|   IBIS model for TI xxx DSP
[IBIS Ver]   5.1
[Disclaimer]   Please be aware that in the absence of a written agreement
|   Texas Instruments(TI) assumes no liability for:
|   (1) The accuracy of the IBIS models provided to your company,
|   however, the IBIS model is compliant to industry standard
|   IQ Level 2a.  Refer to IBIS Quality Section below for
|   for full details.
|   (2) The proper functioning of these Models in your design
|   or for any resulting applications
|   (3) Infringement of patents, copyrights or intellectual
|   property rights resulting from your use of these
|   models.
|   TI provides IBIS Models as a service to our customers and
|   therefore reserves the right to limit distribution of the
|   Models.  The information is subject to change without notice.
[File Name]  sprm825f.ibs
[File Rev]   1.1
|   -Initial version
|   - Removed unsupported SDIO/LVCMOS models
|   - Removed unsupported LVDS models
|   - Removed unsupported IIC and eMMC models
|   - Added LVCMOS models with stronger drive strength supported
|   - Modify default drive strength for EMMC to 50 ohms
|   - Addition of selected drive strengths for EMMC
|   - Addition of power-aware models for eMMC
|   - Updated to align with final AM62P Pkg
|   - Addition of open-drain models for eMMC
|   - Updated to include push-pull models for eMMC
|   - Removed older eMMC models and updated to include models for latest silicon revision
[Date]   16 June 2025
[Source]   Texas Instruments Incorporated
[Copyright]   Property of Texas Instruments Incorporated.
|   Unauthorized reproduction and/or distribution is strictly.
|   prohibited.
|   This product is protected under copyright law and trade
|   secret law as an unpublished work.
|   Created 2012,(C) Copyright 1999-2012,
|   Texas Instruments Incorporated., All Rights Reserved.
|   These commodities are under the U.S. Government
|   distribution license control. As such,they are not to be
|   re-exported without the prior approval of the U.S.
|   Department of Commerce.
[Notes]
   This file does not include AMI models for SerDes based links.
   For SerDes simulations use Texas Instruments IBIS AMI models
   Some IV curves contain Non monotonic data points.
|   Revision History
|   GERNERAL COMMENT: All IBIS Quality Notes below reflect latest release
|   and version of IBIS File
|   File passes ibischk5.1 and ibischk6 with 0 errors and 287 warnings
|   Component AM62P
[Component] AM62P
[Manufacturer] Texas Instruments
[Package]
|   typ   min   max
R_pkg   0.41053   0.082407   0.73268
L_pkg   2.874e-9   9.307e-10   4.887e-9
C_pkg   1.029e-12   4.145e-13   1.599e-12
[Package Model]   am62p_pkg
[Pin]	Signal_name	model_name
B5	ATEST0	NC
Y19	ATEST1	NC
Y13	CSI0_ATB_0_H	NC
Y14	CSI0_ATB_1_H	NC
AE12	CSI0_RXCLKN	NC
AE11	CSI0_RXCLKP	NC
AB11	CSI0_RXN0	NC
AC10	CSI0_RXN1	NC
AA10	CSI0_RXN2	NC
AD9	CSI0_RXN3	NC
AB10	CSI0_RXP0	NC
AC9	CSI0_RXP1	NC
AA9	CSI0_RXP2	NC
AD8	CSI0_RXP3	NC
AA15	CSI0_RXRCALIB	NC
K5	DDR0_A0	DDR_SE
L2	DDR0_A1	DDR_SE
R2	DDR0_A10	DDR_SE
N5	DDR0_A11	DDR_SE
P3	DDR0_A12	DDR_SE
P2	DDR0_A13	DDR_SE
L3	DDR0_A2	DDR_SE
M2	DDR0_A3	DDR_SE
N2	DDR0_A4	DDR_SE
K2	DDR0_A5	DDR_SE
N3	DDR0_A6	DDR_SE
L1	DDR0_A7	DDR_SE
M1	DDR0_A8	DDR_SE
T2	DDR0_A9	DDR_SE
T6	DDR0_ACT_N	DDR_SE
K3	DDR0_ALERT_N	DDR_SE
H5	DDR0_ATB0	DDR_SE
K6	DDR0_ATB1	DDR_SE
N6	DDR0_BA0	DDR_SE
K4	DDR0_BA1	DDR_SE
Y6	DDR0_BG0	DDR_SE
U6	DDR0_BG1	DDR_SE
Y5	DDR0_CAL0	DDR_SE
T5	DDR0_CAS_N	DDR_SE
R1	DDR0_CK0	DDR_DIFF_P
P1	DDR0_CK0_N	DDR_DIFF_N
N4	DDR0_CKE0	DDR_SE
P5	DDR0_CKE1	DDR_SE
L6	DDR0_CS0_N	DDR_SE
T3	DDR0_CS1_N	DDR_SE
C3	DDR0_DM0	DDR_SE
H3	DDR0_DM1	DDR_SE
V4	DDR0_DM2	DDR_SE
AD1	DDR0_DM3	DDR_SE
B2	DDR0_DQ0	DDR_SE
A3	DDR0_DQ1	DDR_SE
G5	DDR0_DQ10	DDR_SE
F2	DDR0_DQ11	DDR_SE
G3	DDR0_DQ12	DDR_SE
H4	DDR0_DQ13	DDR_SE
J2	DDR0_DQ14	DDR_SE
G2	DDR0_DQ15	DDR_SE
U2	DDR0_DQ16	DDR_SE
U3	DDR0_DQ17	DDR_SE
U5	DDR0_DQ18	DDR_SE
V5	DDR0_DQ19	DDR_SE
A4	DDR0_DQ2	DDR_SE
V2	DDR0_DQ20	DDR_SE
Y2	DDR0_DQ21	DDR_SE
Y3	DDR0_DQ22	DDR_SE
AA4	DDR0_DQ23	DDR_SE
AC2	DDR0_DQ24	DDR_SE
AA2	DDR0_DQ25	DDR_SE
AC4	DDR0_DQ26	DDR_SE
AD2	DDR0_DQ27	DDR_SE
AD3	DDR0_DQ28	DDR_SE
AC3	DDR0_DQ29	DDR_SE
A5	DDR0_DQ3	DDR_SE
AE4	DDR0_DQ30	DDR_SE
AE3	DDR0_DQ31	DDR_SE
A2	DDR0_DQ4	DDR_SE
B4	DDR0_DQ5	DDR_SE
D2	DDR0_DQ6	DDR_SE
C4	DDR0_DQ7	DDR_SE
E2	DDR0_DQ8	DDR_SE
F1	DDR0_DQ9	DDR_SE
D1	DDR0_DQS0	DDR_DIFF_P
C1	DDR0_DQS0_N	DDR_DIFF_N
J1	DDR0_DQS1	DDR_DIFF_P
H1	DDR0_DQS1_N	DDR_DIFF_N
W1	DDR0_DQS2	DDR_DIFF_P
V1	DDR0_DQS2_N	DDR_DIFF_N
AA1	DDR0_DQS3	DDR_DIFF_P
AB1	DDR0_DQS3_N	DDR_DIFF_N
L5	DDR0_ODT0	DDR_SE
V6	DDR0_ODT1	DDR_SE
T1	DDR0_PAR	DDR_SE
P6	DDR0_RAS_N	DDR_SE
AA5	DDR0_RESET0_N	DDR_SE
T4	DDR0_WE_N	DDR_SE
AA17	DSI0_ATB_0_H	NC
Y17	DSI0_ATB_1_H	NC
AA12	DSI0_TXCLKN	NC
AA13	DSI0_TXCLKP	NC
AD11	DSI0_TXN0	NC
AB13	DSI0_TXN1	NC
AC12	DSI0_TXN2	NC
AE14	DSI0_TXN3	NC
AD12	DSI0_TXP0	NC
AB14	DSI0_TXP1	NC
AC13	DSI0_TXP2	NC
AE15	DSI0_TXP3	NC
Y16	DSI0_TXRCALIB	NC
B12	EMU0	LVCMOS_V
D13	EMU1	LVCMOS_V
C25	EXT_REFCLK1	LVCMOS_V
C23	EXTINTN	IIC_V
U22	GPMC0_AD0	LVCMOS_H
U21	GPMC0_AD1	LVCMOS_H
AA25	GPMC0_AD10	LVCMOS_H
W24	GPMC0_AD11	LVCMOS_H
Y24	GPMC0_AD12	LVCMOS_H
AD25	GPMC0_AD13	LVCMOS_H
AB24	GPMC0_AD14	LVCMOS_H
AC24	GPMC0_AD15	LVCMOS_H
U20	GPMC0_AD2	LVCMOS_H
V25	GPMC0_AD3	LVCMOS_H
T20	GPMC0_AD4	LVCMOS_H
T21	GPMC0_AD5	LVCMOS_H
V24	GPMC0_AD6	LVCMOS_H
W25	GPMC0_AD7	LVCMOS_H
AC25	GPMC0_AD8	LVCMOS_H
AB25	GPMC0_AD9	LVCMOS_H
R25	GPMC0_ADVN_ALE	LVCMOS_H
U24	GPMC0_BE0N_CLE	LVCMOS_H
T24	GPMC0_BE1N	LVCMOS_H
Y25	GPMC0_CLK	LVCMOS_H
T23	GPMC0_CSN0	LVCMOS_H
U23	GPMC0_CSN1	LVCMOS_H
T22	GPMC0_CSN2	LVCMOS_H
U25	GPMC0_CSN3	LVCMOS_H
P25	GPMC0_DIR	LVCMOS_H
R24	GPMC0_OEN_REN	LVCMOS_H
AA24	GPMC0_WAIT0	LVCMOS_H
AD24	GPMC0_WAIT1	LVCMOS_H
T25	GPMC0_WEN	LVCMOS_H
P24	GPMC0_WPN	LVCMOS_H
B25	I2C0_SCL	LVCMOS_V
A24	I2C0_SDA	LVCMOS_V
C24	I2C1_SCL	LVCMOS_V
B24	I2C1_SDA	LVCMOS_V
C5	IFORCE	NC
F20	MCAN0_RX	LVCMOS_V
B23	MCAN0_TX	LVCMOS_V
G20	MCASP0_ACLKR	LVCMOS_V
F24	MCASP0_ACLKX	LVCMOS_V
G23	MCASP0_AFSR	LVCMOS_V
F25	MCASP0_AFSX	LVCMOS_V
F23	MCASP0_AXR0	LVCMOS_V
E24	MCASP0_AXR1	LVCMOS_V
E25	MCASP0_AXR2	LVCMOS_V
D25	MCASP0_AXR3	LVCMOS_V
G6	MCU_ERRORN	LVCMOS_H
E11	MCU_I2C0_SCL	IIC_V
D11	MCU_I2C0_SDA	IIC_V
D6	MCU_MCAN0_RX	LVCMOS_V
E8	MCU_MCAN0_TX	LVCMOS_V
E7	MCU_MCAN1_RX	LVCMOS_V
F8	MCU_MCAN1_TX	LVCMOS_V
A10	MCU_OSC0_XI	NC
A11	MCU_OSC0_XO	NC
H6	MCU_PORZ	RESET_H
F14	MCU_RESETSTATZ	LVCMOS_V
F11	MCU_RESETZ	LVCMOS_V
C10	MCU_SPI0_CLK	LVCMOS_V
B10	MCU_SPI0_CS0	LVCMOS_V
E10	MCU_SPI0_CS1	LVCMOS_V
B11	MCU_SPI0_D0	LVCMOS_V
D10	MCU_SPI0_D1	LVCMOS_V
B8	MCU_UART0_CTSN	LVCMOS_V
B7	MCU_UART0_RTSN	LVCMOS_V
B6	MCU_UART0_RXD	LVCMOS_V
C8	MCU_UART0_TXD	LVCMOS_V
F17	MDIO0_MDC	LVCMOS_V
F16	MDIO0_MDIO	LVCMOS_V
AC5	MMC0_CALPAD	EMMC
AA6	MMC0_CLK	EMMC
AB8	MMC0_CMD	EMMC
AC7	MMC0_DAT0	EMMC
AB7	MMC0_DAT1	EMMC
AD6	MMC0_DAT2	EMMC
AE5	MMC0_DAT3	EMMC
AE6	MMC0_DAT4	EMMC
AC6	MMC0_DAT5	EMMC
AA7	MMC0_DAT6	EMMC
AB6	MMC0_DAT7	EMMC
AD5	MMC0_DS	EMMC
J24	MMC1_CLK	SDIO_V
H20	MMC1_CMD	SDIO_V
H21	MMC1_DAT0	SDIO_V
H23	MMC1_DAT1	SDIO_V
H22	MMC1_DAT2	SDIO_V
H25	MMC1_DAT3	SDIO_V
D23	MMC1_SDCD	LVCMOS_V
D24	MMC1_SDWP	LVCMOS_V
K21	MMC2_CLK	SDIO_H
K24	MMC2_CMD	SDIO_H
K23	MMC2_DAT0	SDIO_H
K22	MMC2_DAT1	SDIO_H
L20	MMC2_DAT2	SDIO_H
L21	MMC2_DAT3	SDIO_H
J25	MMC2_SDCD	LVCMOS_H
K25	MMC2_SDWP	LVCMOS_H
AE20	OLDI0_A0N	LVDS
AD20	OLDI0_A0P	LVDS
AC19	OLDI0_A1N	LVDS
AD19	OLDI0_A1P	LVDS
AA19	OLDI0_A2N	LVDS
AB19	OLDI0_A2P	LVDS
AD18	OLDI0_A3N	LVDS
AE19	OLDI0_A3P	LVDS
AD17	OLDI0_A4N	LVDS
AD16	OLDI0_A4P	LVDS
AB17	OLDI0_A5N	LVDS
AC17	OLDI0_A5P	LVDS
AC16	OLDI0_A6N	LVDS
AC15	OLDI0_A6P	LVDS
AB16	OLDI0_A7N	LVDS
AA16	OLDI0_A7P	LVDS
AE18	OLDI0_CLK0N	LVDS
AE17	OLDI0_CLK0P	LVDS
AD15	OLDI0_CLK1N	LVDS
AD14	OLDI0_CLK1P	LVDS
P23	OSPI0_CLK	LVCMOS_H
M25	OSPI0_CSN0	LVCMOS_H
L24	OSPI0_CSN1	LVCMOS_H
L22	OSPI0_CSN2	LVCMOS_H
L23	OSPI0_CSN3	LVCMOS_H
L25	OSPI0_D0	LVCMOS_H
N24	OSPI0_D1	LVCMOS_H
N25	OSPI0_D2	LVCMOS_H
M24	OSPI0_D3	LVCMOS_H
N21	OSPI0_D4	LVCMOS_H
N22	OSPI0_D5	LVCMOS_H
P21	OSPI0_D6	LVCMOS_H
N20	OSPI0_D7	LVCMOS_H
P22	OSPI0_DQS	LVCMOS_H
N23	OSPI0_LBCLKO	LVCMOS_H
B9	PMIC_LPM_EN0	LVCMOS_V
H24	PORZ_OUT	LVCMOS_V
G24	RESET_REQZ	LVCMOS_V
G25	RESETSTATZ	LVCMOS_V
B15	RGMII1_RD0	LVCMOS_V
B16	RGMII1_RD1	LVCMOS_V
A14	RGMII1_RD2	LVCMOS_V
B14	RGMII1_RD3	LVCMOS_V
A15	RGMII1_RX_CTL	LVCMOS_V
A16	RGMII1_RXC	LVCMOS_V
A18	RGMII1_TD0	LVCMOS_V
C17	RGMII1_TD1	LVCMOS_V
A17	RGMII1_TD2	LVCMOS_V
C16	RGMII1_TD3	LVCMOS_V
B18	RGMII1_TX_CTL	LVCMOS_V
B17	RGMII1_TXC	LVCMOS_V
E19	RGMII2_RD0	LVCMOS_V
E16	RGMII2_RD1	LVCMOS_V
E17	RGMII2_RD2	LVCMOS_V
C19	RGMII2_RD3	LVCMOS_V
F19	RGMII2_RX_CTL	LVCMOS_V
D19	RGMII2_RXC	LVCMOS_V
B19	RGMII2_TD0	LVCMOS_V
A21	RGMII2_TD1	LVCMOS_V
D17	RGMII2_TD2	LVCMOS_V
A19	RGMII2_TD3	LVCMOS_V
A20	RGMII2_TX_CTL	LVCMOS_V
D16	RGMII2_TXC	LVCMOS_V
B21	SPI0_CLK	LVCMOS_V
D20	SPI0_CS0	LVCMOS_V
E20	SPI0_CS1	LVCMOS_V
B20	SPI0_D0	LVCMOS_V
C21	SPI0_D1	LVCMOS_V
C13	TCK	LVCMOS_V
E13	TDI	LVCMOS_V
C14	TDO	LVCMOS_V
F10	TEMP_DIODE_P	NC
E14	TMS	LVCMOS_V
B13	TRSTN	LVCMOS_V
A23	UART0_CTSN	LVCMOS_V
C22	UART0_RTSN	LVCMOS_V
A22	UART0_RXD	LVCMOS_V
B22	UART0_TXD	LVCMOS_V
AE8	USB0_DM	NC
AE7	USB0_DP	NC
G22	USB0_DRVVBUS	LVCMOS_V
Y8	USB0_RCALIB	NC
Y7	USB0_VBUS	NC
AE10	USB1_DM	NC
AE9	USB1_DP	NC
G21	USB1_DRVVBUS	LVCMOS_V
1K4	USB1_RCALIB	NC
Y10	USB1_VBUS	NC
1A10	VMON_1P8_SOC	NC
1A4	VMON_3P3_SOC	NC
1A6	VMON_ER_VSYS	NC
AE24	VOUT0_DATA0	LVCMOS_H
W23	VOUT0_DATA1	LVCMOS_H
W22	VOUT0_DATA10	LVCMOS_H
AE21	VOUT0_DATA11	LVCMOS_H
AD21	VOUT0_DATA12	LVCMOS_H
AC21	VOUT0_DATA13	LVCMOS_H
AA20	VOUT0_DATA14	LVCMOS_H
Y20	VOUT0_DATA15	LVCMOS_H
AA23	VOUT0_DATA2	LVCMOS_H
Y23	VOUT0_DATA3	LVCMOS_H
AB23	VOUT0_DATA4	LVCMOS_H
AD23	VOUT0_DATA5	LVCMOS_H
AC23	VOUT0_DATA6	LVCMOS_H
AE23	VOUT0_DATA7	LVCMOS_H
AE22	VOUT0_DATA8	LVCMOS_H
AC22	VOUT0_DATA9	LVCMOS_H
W21	VOUT0_DE	LVCMOS_H
AC20	VOUT0_HSYNC	LVCMOS_H
Y21	VOUT0_PCLK	LVCMOS_H
W20	VOUT0_VSYNC	LVCMOS_H
F6	VSENSE	NC
F13	WKUP_CLKOUT0	LVCMOS_V
A13	WKUP_I2C0_SCL	IIC_V
C11	WKUP_I2C0_SDA	IIC_V
A7	WKUP_LFOSC0_XI	NC
A8	WKUP_LFOSC0_XO	NC
C7	WKUP_UART0_CTSN	LVCMOS_V
C6	WKUP_UART0_RTSN	LVCMOS_V
D8	WKUP_UART0_RXD	LVCMOS_V
D7	WKUP_UART0_TXD	LVCMOS_V
A1	VSS	GND
A6	VSS	GND
A9	VSS	GND
A12	VSS	GND
A25	VSS	GND
1G1	VSS	GND
1G4	VSS	GND
1G6	VSS	GND
1G8	VSS	GND
1H2	VSS	GND
1H5	VSS	GND
1H9	VSS	GND
1J3	VSS	GND
1J6	VSS	GND
1J8	VSS	GND
1J10	VSS	GND
U1	VSS	GND
U4	VSS	GND
1K1	VSS	GND
1K9	VSS	GND
V3	VSS	GND
W2	VSS	GND
Y1	VSS	GND
Y4	VSS	GND
AA3	VSS	GND
AA21	VSS	GND
AB2	VSS	GND
AC1	VSS	GND
AD4	VSS	GND
AD22	VSS	GND
AE1	VSS	GND
AE13	VSS	GND
AE16	VSS	GND
AE25	VSS	GND
B3	VSS	GND
C2	VSS	GND
C20	VSS	GND
D3	VSS	GND
D14	VSS	GND
E1	VSS	GND
F3	VSS	GND
G1	VSS	GND
G4	VSS	GND
H2	VSS	GND
1A3	VSS	GND
1A5	VSS	GND
1A7	VSS	GND
1B1	VSS	GND
1B8	VSS	GND
K1	VSS	GND
1C4	VSS	GND
1C6	VSS	GND
L4	VSS	GND
1D1	VSS	GND
1D5	VSS	GND
1D9	VSS	GND
1E4	VSS	GND
1E6	VSS	GND
1E8	VSS	GND
N1	VSS	GND
1F3	VSS	GND
1F7	VSS	GND
1F9	VSS	GND
P4	VSS	GND
P20	VSS	GND
1A8	CAP_VDDS0		POWER
1C10	CAP_VDDS1   POWER
1B6	CAP_VDDS2   POWER
1F10	CAP_VDDS3   POWER
1B9   CAP_VDDS5   POWER
1C9 	CAP_VDDS6   POWER
1B2 	CAP_VDDS_CANUART	POWER
1B4 	CAP_VDDS_MCU		POWER
1K7 	VDDA_1P8_CSI_DSI	POWER
1K10	VDDA_1P8_OLDI0		POWER
1K5 	VDDA_1P8_USB		POWER
Y11 	VDDA_3P3_USB 		POWER
1K6   VDDA_CORE_CSI_DSI 	POWER
1K8  	VDDA_CORE_DSI_CLK  	POWER
1J4   VDDA_CORE_USB   POWER
1F2   VDDA_DDR_PLL0   POWER
1C3   VDDA_MCU   POWER
1D4 	VDDA_PLL0   POWER
1H7 	VDDA_PLL1   POWER
1F6 	VDDA_PLL2   POWER
1F4	VDDA_PLL3   POWER
1D7	VDDA_PLL4		POWER
1F5	VDDA_TEMP0 		POWER
K20	VDDA_TEMP1		POWER
1D3	VDDA_TEMP2   POWER
1C8 	VDDR_CORE   POWER
1E5	VDDR_CORE   POWER
1H3 	VDDR_CORE   POWER
1J1	VDDR_CORE 		POWER
1K3 	VDDR_CORE   POWER
1B7	VDDSHV0   POWER
1D10	VDDSHV1   POWER
1B5	VDDSHV2   POWER
1E10	VDDSHV3   POWER
1G10	VDDSHV3   POWER
1A9 	VDDSHV5   POWER
1B10	VDDSHV6   POWER
1A2   VDDSHV_CANUART   POWER
1B3 	VDDSHV_MCU   POWER
1C1	VDDS_DDR   POWER
1D2 	VDDS_DDR   POWER
1E1	VDDS_DDR   POWER
1F1	VDDS_DDR   POWER
1G2 	VDDS_DDR   POWER
1H1  	VDDS_DDR   POWER
AE2 	VDDS_DDR   POWER
B1	VDDS_DDR   POWER
1E2 	VDDS_DDR_C   POWER
1K2 	VDDS_MMC0 		POWER
1C2	VDDS_OSC0   POWER
1A1 	VDD_CANUART 		POWER
1C5	VDD_CORE   POWER
1C7  	VDD_CORE   POWER
1D6 	VDD_CORE		POWER
1D8	VDD_CORE		POWER
1E3	VDD_CORE		POWER
1E7	VDD_CORE		POWER
1E9	VDD_CORE		POWER
1F8	VDD_CORE		POWER
1G3	VDD_CORE		POWER
1G5	VDD_CORE		POWER
1G7	VDD_CORE		POWER
1G9	VDD_CORE		POWER
1H4	VDD_CORE		POWER
1H6	VDD_CORE		POWER
1H8	VDD_CORE		POWER
1H10	VDD_CORE		POWER
1J2	VDD_CORE		POWER
1J5	VDD_CORE		POWER
1J7	VDD_CORE		POWER
1J9	VDD_CORE		POWER
F7	VPP			POWER
|********************  DIFF PIN  *******************************
[Diff_pin]   inv_pin vdiff tdelay_typ   tdelay_min  tdelay_max
R1	P1	NA	NA	NA	NA	||	DDR0_CK0	&	DDR0_CK0_N
D1	C1	NA	NA	NA	NA	||	DDR0_DQS0	&	DDR0_DQS0_N
J1	H1	NA	NA	NA	NA	||	DDR0_DQS1	&	DDR0_DQS1_N
W1	V1	NA	NA	NA	NA	||	DDR0_DQS2	&	DDR0_DQS2_N
AA1	AB1	NA	NA	NA	NA	||	DDR0_DQS3	&	DDR0_DQS3_N
AE20	AD20	NA	NA	NA	NA	||	OLDI0_A0N	&	OLDI0_A0P
AC19	AD19	NA	NA	NA	NA	||	OLDI0_A1N	&	OLDI0_A1P
AA19	AB19	NA	NA	NA	NA	||	OLDI0_A2N	&	OLDI0_A2P
AD18	AE19	NA	NA	NA	NA	||	OLDI0_A3N	&	OLDI0_A3P
AD17	AD16	NA	NA	NA	NA	||	OLDI0_A4N	&	OLDI0_A4P
AB17	AC17	NA	NA	NA	NA	||	OLDI0_A5N	&	OLDI0_A5P
AC16	AC15	NA	NA	NA	NA	||	OLDI0_A6N	&	OLDI0_A6P
AB16	AA16	NA	NA	NA	NA	||	OLDI0_A7N	&	OLDI0_A7P
AE18	AE17	NA	NA	NA	NA	||	OLDI0_CLK0N	&	OLDI0_CLK0P
AD15	AD14	NA	NA	NA	NA	||	OLDI0_CLK1N	&	OLDI0_CLK1P
|---------------- DDR -------------------
[Model Selector] DDR_SE
lpddr4_ocd_40p_40n_lt  driver with 40 ohms pullup and 40 ohms pulldown strength, max slew rate
lpddr4_ocd_48p_48n_lt  driver with 48 ohms pullup and 48 ohms pulldown strength, max slew rate
lpddr4_ocd_60p_60n_lt  driver with 60 ohms pullup and 60 ohms pulldown strength, max slew rate
lpddr4_ocd_60p_60n_120pd_lt  driver with 60 ohms pd and 60 ohms pu and 120 pd always on, max slew rate
lpddr4_ocd_80p_80n_lt  driver with 80 ohms pullup and 80 ohms pulldown strength, max slew rate
lpddr4_odt_40_lt  40 ohm termination
lpddr4_odt_48_lt  48 ohm termination
lpddr4_odt_60_lt  60 ohm termination
lpddr4_odt_80_lt  80 ohm termination
lpddr4_odt_120_lt  120 ohm termination
lpddr4_odt_240_lt  240 ohm termination
lpddr4_odt_off_lt  No termination
ddr4_ocd_34p_34n_lt  driver with 34 ohms pullup and 34 ohms pulldown strength, max slew rate
ddr4_ocd_40p_40n_lt  driver with 40 ohms pullup and 40 ohms pulldown strength, max slew rate
ddr4_ocd_48p_48n_lt  driver with 48 ohms pullup and 48 ohms pulldown strength, max slew rate
ddr4_ocd_60p_60n_lt  driver with 60 ohms pullup and 60 ohms pulldown strength, max slew rate
ddr4_ocd_80p_80n_lt  driver with 80 ohms pullup and 80 ohms pulldown strength, max slew rate
ddr4_odt_34_lt  34 ohm termination
ddr4_odt_40_lt  40 ohm termination
ddr4_odt_48_lt  48 ohm termination
ddr4_odt_60_lt  60 ohm termination
ddr4_odt_80_lt  80 ohm termination
ddr4_odt_120_lt  120 ohm termination
ddr4_odt_240_lt  240 ohm termination
ddr4_odt_off_lt  No termination
lpddr4_ocd_40p_40n_ht  driver with 40 ohms pullup and 40 ohms pulldown strength, max slew rate
lpddr4_ocd_48p_48n_ht  driver with 48 ohms pullup and 48 ohms pulldown strength, max slew rate
lpddr4_ocd_60p_60n_ht  driver with 60 ohms pullup and 60 ohms pulldown strength, max slew rate
lpddr4_ocd_60p_60n_120pd_ht  driver with 60 ohms pd and 60 ohms pu and 120 pd always on, max slew rate
lpddr4_ocd_80p_80n_ht  driver with 80 ohms pullup and 80 ohms pulldown strength, max slew rate
lpddr4_odt_40_ht  40 ohm termination
lpddr4_odt_48_ht  48 ohm termination
lpddr4_odt_60_ht  60 ohm termination
lpddr4_odt_80_ht  80 ohm termination
lpddr4_odt_120_ht  120 ohm termination
lpddr4_odt_240_ht  240 ohm termination
lpddr4_odt_off_ht  No termination
ddr4_ocd_34p_34n_ht  driver with 34 ohms pullup and 34 ohms pulldown strength, max slew rate
ddr4_ocd_40p_40n_ht  driver with 40 ohms pullup and 40 ohms pulldown strength, max slew rate
ddr4_ocd_48p_48n_ht  driver with 48 ohms pullup and 48 ohms pulldown strength, max slew rate
ddr4_ocd_60p_60n_ht  driver with 60 ohms pullup and 60 ohms pulldown strength, max slew rate
ddr4_ocd_80p_80n_ht  driver with 80 ohms pullup and 80 ohms pulldown strength, max slew rate
ddr4_odt_34_ht  34 ohm termination
ddr4_odt_40_ht  40 ohm termination
ddr4_odt_48_ht  48 ohm termination
ddr4_odt_60_ht  60 ohm termination
ddr4_odt_80_ht  80 ohm termination
ddr4_odt_120_ht  120 ohm termination
ddr4_odt_240_ht  240 ohm termination
ddr4_odt_off_ht  No termination
[Model Selector] DDR_DIFF_P
lpddr4_ocd_40p_40n_p_lt  driver with 40 ohms pullup and 40 ohms pulldown strength, max slew rate
lpddr4_ocd_48p_48n_p_lt  driver with 48 ohms pullup and 48 ohms pulldown strength, max slew rate
lpddr4_ocd_60p_60n_p_lt  driver with 60 ohms pullup and 60 ohms pulldown strength, max slew rate
lpddr4_ocd_60p_60n_120pd_p_lt  driver with 60 ohms pd and 60 ohms pu and 120 pd always on, max slew rate
lpddr4_ocd_80p_80n_p_lt  driver with 80 ohms pullup and 80 ohms pulldown strength, max slew rate
lpddr4_odt_40_diff_lt  40 ohm termination
lpddr4_odt_48_diff_lt  48 ohm termination
lpddr4_odt_60_diff_lt  60 ohm termination
lpddr4_odt_80_diff_lt  80 ohm termination
lpddr4_odt_120_diff_lt  120 ohm termination
lpddr4_odt_240_diff_lt  240 ohm termination
lpddr4_odt_off_diff_lt  No termination
ddr4_ocd_34p_34n_P_lt  driver with 34 ohms pullup and 34 ohms pulldown strength, max slew rate
ddr4_ocd_40p_40n_P_lt  driver with 40 ohms pullup and 40 ohms pulldown strength, max slew rate
ddr4_ocd_48p_48n_P_lt  driver with 48 ohms pullup and 48 ohms pulldown strength, max slew rate
ddr4_ocd_60p_60n_P_lt  driver with 60 ohms pullup and 60 ohms pulldown strength, max slew rate
ddr4_ocd_80p_80n_P_lt  driver with 80 ohms pullup and 80 ohms pulldown strength, max slew rate
ddr4_odt_34_diff_lt  34 ohm termination
ddr4_odt_40_diff_lt  40 ohm termination
ddr4_odt_48_diff_lt  48 ohm termination
ddr4_odt_60_diff_lt  60 ohm termination
ddr4_odt_80_diff_lt  80 ohm termination
ddr4_odt_120_diff_lt  120 ohm termination
ddr4_odt_240_diff_lt  240 ohm termination
ddr4_odt_off_diff_lt  No termination
lpddr4_ocd_40p_40n_p_ht  driver with 40 ohms pullup and 40 ohms pulldown strength, max slew rate
lpddr4_ocd_48p_48n_p_ht  driver with 48 ohms pullup and 48 ohms pulldown strength, max slew rate
lpddr4_ocd_60p_60n_p_ht  driver with 60 ohms pullup and 60 ohms pulldown strength, max slew rate
lpddr4_ocd_60p_60n_120pd_p_ht  driver with 60 ohms pd and 60 ohms pu and 120 pd always on, max slew rate
lpddr4_ocd_80p_80n_p_ht  driver with 80 ohms pullup and 80 ohms pulldown strength, max slew rate
lpddr4_odt_40_diff_ht  40 ohm termination
lpddr4_odt_48_diff_ht  48 ohm termination
lpddr4_odt_60_diff_ht  60 ohm termination
lpddr4_odt_80_diff_ht  80 ohm termination
lpddr4_odt_120_diff_ht  120 ohm termination
lpddr4_odt_240_diff_ht  240 ohm termination
lpddr4_odt_off_diff_ht  No termination
ddr4_ocd_34p_34n_P_ht  driver with 34 ohms pullup and 34 ohms pulldown strength, max slew rate
ddr4_ocd_40p_40n_P_ht  driver with 40 ohms pullup and 40 ohms pulldown strength, max slew rate
ddr4_ocd_48p_48n_P_ht  driver with 48 ohms pullup and 48 ohms pulldown strength, max slew rate
ddr4_ocd_60p_60n_P_ht  driver with 60 ohms pullup and 60 ohms pulldown strength, max slew rate
ddr4_ocd_80p_80n_P_ht  driver with 80 ohms pullup and 80 ohms pulldown strength, max slew rate
ddr4_odt_34_diff_ht  34 ohm termination
ddr4_odt_40_diff_ht  40 ohm termination
ddr4_odt_48_diff_ht  48 ohm termination
ddr4_odt_60_diff_ht  60 ohm termination
ddr4_odt_80_diff_ht  80 ohm termination
ddr4_odt_120_diff_ht  120 ohm termination
ddr4_odt_240_diff_ht  240 ohm termination
ddr4_odt_off_diff_ht  No termination
[Model Selector] DDR_DIFF_N
lpddr4_ocd_40p_40n_n_lt  driver with 40 ohms pullup and 40 ohms pulldown strength, max slew rate
lpddr4_ocd_48p_48n_n_lt  driver with 48 ohms pullup and 48 ohms pulldown strength, max slew rate
lpddr4_ocd_60p_60n_n_lt  driver with 60 ohms pullup and 60 ohms pulldown strength, max slew rate
lpddr4_ocd_60p_60n_120pd_n_lt  driver with 60 ohms pd and 60 ohms pu and 120 pd always on, max slew rate
lpddr4_ocd_80p_80n_n_lt  driver with 80 ohms pullup and 80 ohms pulldown strength, max slew rate
lpddr4_odt_40_diff_lt  40 ohm termination
lpddr4_odt_48_diff_lt  48 ohm termination
lpddr4_odt_60_diff_lt  60 ohm termination
lpddr4_odt_80_diff_lt  80 ohm termination
lpddr4_odt_120_diff_lt  120 ohm termination
lpddr4_odt_240_diff_lt  240 ohm termination
lpddr4_odt_off_diff_lt  No termination
ddr4_ocd_34p_34n_N_lt  driver with 34 ohms pullup and 34 ohms pulldown strength, max slew rate
ddr4_ocd_40p_40n_N_lt  driver with 40 ohms pullup and 40 ohms pulldown strength, max slew rate
ddr4_ocd_48p_48n_N_lt  driver with 48 ohms pullup and 48 ohms pulldown strength, max slew rate
ddr4_ocd_60p_60n_N_lt  driver with 60 ohms pullup and 60 ohms pulldown strength, max slew rate
ddr4_ocd_80p_80n_N_lt  driver with 80 ohms pullup and 80 ohms pulldown strength, max slew rate
ddr4_odt_34_diff_lt  34 ohm termination
ddr4_odt_40_diff_lt  40 ohm termination
ddr4_odt_48_diff_lt  48 ohm termination
ddr4_odt_60_diff_lt  60 ohm termination
ddr4_odt_80_diff_lt  80 ohm termination
ddr4_odt_120_diff_lt  120 ohm termination
ddr4_odt_240_diff_lt  240 ohm termination
ddr4_odt_off_diff_lt  No termination
lpddr4_ocd_40p_40n_n_ht  driver with 40 ohms pullup and 40 ohms pulldown strength, max slew rate
lpddr4_ocd_48p_48n_n_ht  driver with 48 ohms pullup and 48 ohms pulldown strength, max slew rate
lpddr4_ocd_60p_60n_n_ht  driver with 60 ohms pullup and 60 ohms pulldown strength, max slew rate
lpddr4_ocd_60p_60n_120pd_n_ht  driver with 60 ohms pd and 60 ohms pu and 120 pd always on, max slew rate
lpddr4_ocd_80p_80n_n_ht  driver with 80 ohms pullup and 80 ohms pulldown strength, max slew rate
lpddr4_odt_40_diff_ht  40 ohm termination
lpddr4_odt_48_diff_ht  48 ohm termination
lpddr4_odt_60_diff_ht  60 ohm termination
lpddr4_odt_80_diff_ht  80 ohm termination
lpddr4_odt_120_diff_ht  120 ohm termination
lpddr4_odt_240_diff_ht  240 ohm termination
lpddr4_odt_off_diff_ht  No termination
ddr4_ocd_34p_34n_N_ht  driver with 34 ohms pullup and 34 ohms pulldown strength, max slew rate
ddr4_ocd_40p_40n_N_ht  driver with 40 ohms pullup and 40 ohms pulldown strength, max slew rate
ddr4_ocd_48p_48n_N_ht  driver with 48 ohms pullup and 48 ohms pulldown strength, max slew rate
ddr4_ocd_60p_60n_N_ht  driver with 60 ohms pullup and 60 ohms pulldown strength, max slew rate
ddr4_ocd_80p_80n_N_ht  driver with 80 ohms pullup and 80 ohms pulldown strength, max slew rate
ddr4_odt_34_diff_ht  34 ohm termination
ddr4_odt_40_diff_ht  40 ohm termination
ddr4_odt_48_diff_ht  48 ohm termination
ddr4_odt_60_diff_ht  60 ohm termination
ddr4_odt_80_diff_ht  80 ohm termination
ddr4_odt_120_diff_ht  120 ohm termination
ddr4_odt_240_diff_ht  240 ohm termination
ddr4_odt_off_diff_ht  No termination
|****************** SDIO
[Model Selector] SDIO_H
sdio1_r40_1p8_h PRWDWUWSWEWCDGSDIO_H@_R40_1p8_comment
sdio1_r40_3p3_h PRWDWUWSWEWCDGSDIO_H@_R40_3p3_comment
[Model Selector] SDIO_V
sdio0_r40_1p8_v PRWDWUWSWEWCDGSDIO_V@_R40_1p8_comment
sdio0_r40_3p3_v PRWDWUWSWEWCDGSDIO_V@_R40_3p3_comment
|********** LVCMOS
[Model Selector] LVCMOS_H
lvcmos1_nom_1p8_h PRWDWUWSWEWCDGLVCMOS_H@_Nom_1p8_comment
lvcmos1_nom_3p3_h PRWDWUWSWEWCDGLVCMOS_H@_Nom_3p3_comment
lvcmos1_fast_1p8_h PRWDWUWSWEWCDGLVCMOS_H@_Fast_1p8_comment
lvcmos1_fast_3p3_h PRWDWUWSWEWCDGLVCMOS_H@_Fast_3p3_comment
[Model Selector] LVCMOS_V
lvcmos0_nom_1p8_v PRWDWUWSWEWCDGLVCMOS_V@_Nom_1p8_comment
lvcmos0_nom_3p3_v PRWDWUWSWEWCDGLVCMOS_V@_Nom_3p3_comment
lvcmos0_fast_1p8_v PRWDWUWSWEWCDGLVCMOS_V@_Fast_1p8_comment
lvcmos0_fast_3p3_v PRWDWUWSWEWCDGLVCMOS_V@_Fast_3p3_comment
[Model Selector] IIC_V
IIC18_1_0_V PRBOPDDGZIIC_V@HSMODE_HSMCSE=0_0_comment 1.8V
IIC18_1_1_V PRBOPDDGZIIC_V@HSMODE_HSMCSE=0_1_comment 1.8V
IIC18_1_2_V PRBOPDDGZIIC_V@HSMODE_HSMCSE=1_0_comment 1.8V
IIC18_1_3_V PRBOPDDGZIIC_V@HSMODE_HSMCSE=1_1_comment 1.8V
IIC33_1_0_V PRBOPDDGZIIC_V@HSMODE_HSMCSE=0_0_comment
[Model Selector] LVDS
lvds_tx_03   LVDS TX Driver Permumentation 03
lvds_tx_11   LVDS TX Driver Permumentation 11
|***************** RESET ************************************************
[Model Selector] RESET_H
reset18_0_0 PDIDGZRESET_H
|   EMMC
[MODEL SELECTOR] EMMC
emmc51_io_000   50ohm DRIVE  I/O model when dr_ty[2]=0 ,dr_ty[1]=0 ,dr_ty[0]=0
emmc51_io_001   33ohm DRIVE  I/O model when dr_ty[2]=0 ,dr_ty[1]=0 ,dr_ty[0]=1
emmc51_io_010   66ohm DRIVE  I/O model when dr_ty[2]=0 ,dr_ty[1]=1 ,dr_ty[0]=0
emmc51_io_100   40ohm DRIVE  I/O model when dr_ty[2]=1 ,dr_ty[1]=0 ,dr_ty[0]=0
io_od_1p8_000   50ohm  I/O_open_drain model
io_od_1p8_001   33ohm  I/O_open_drain model
io_od_1p8_010   66ohm  I/O_open_drain model
io_od_1p8_100   40ohm  I/O_open_drain model
|   Package Model
[Define Package Model]   am62p_pkg
[Manufacturer]   name 1
[OEM]   name 2
[Description]   370-pin Package
|[Number of Sections]   1
[Number of Pins]   370
[Pin Numbers]
|[Pin Name]  Net Number   Net Name   Net's All Pins
1A8   | 1   CAP_VDDS0   1A8
1C10   | 2   CAP_VDDS1   1C10
1B6   | 3   CAP_VDDS2   1B6
1F10   | 4   CAP_VDDS3   1F10
1B9   | 5   CAP_VDDS5   1B9
1C9   | 6   CAP_VDDS6   1C9
1B2   | 7   CAP_VDDS_CANUART   1B2
1B4   | 8   CAP_VDDS_MCU   1B4
1K7   | 9   VDDA_1P8_CSI_DSI   1K7
1K10   | 10   VDDA_1P8_OLDI0   1K10
1K5   | 11   VDDA_1P8_USB   1K5
Y11   | 12   VDDA_3P3_USB   Y11
1K6   | 13   VDDA_CORE_CSI_DSI   1K6
1K8   | 14   VDDA_CORE_DSI_CLK   1K8
1J4   | 15   VDDA_CORE_USB   1J4
1F2   | 16   VDDA_DDR_PLL0   1F2
1C3   | 17   VDDA_MCU   1C3
1D4   | 18   VDDA_PLL0   1D4
1H7   | 19   VDDA_PLL1   1H7
1F6   | 20   VDDA_PLL2   1F6
1F4   | 21   VDDA_PLL3   1F4
1D7   | 22   VDDA_PLL4   1D7
1F5   | 23   VDDA_TEMP0   1F5
K20   | 24   VDDA_TEMP1   K20
1D3   | 25   VDDA_TEMP2   1D3
1C8   | 26   VDDR_CORE   1C8
   |1E5
   |1H3
   |1J1
   |1K3
1B7   | 27   VDDSHV0   1B7
1D10   | 28   VDDSHV1   1D10
1B5   | 29   VDDSHV2   1B5
1E10   | 30   VDDSHV3   1E10
   |1G10
1A9   | 31   VDDSHV5   1A9
1B10   | 32   VDDSHV6   1B10
1A2   | 33   VDDSHV_CANUART   1A2
1B3   | 34   VDDSHV_MCU   1B3
1C1   | 35   VDDS_DDR   1C1
   |1D2
   |1E1
   |1F1
   |1G2
   |1H1
   |AE2
   |B1
1E2   | 36   VDDS_DDR_C   1E2
1K2   | 37   VDDS_MMC0   1K2
1C2   | 38   VDDS_OSC0   1C2
1A1   | 39   VDD_CANUART   1A1
1C5   | 40   VDD_CORE   1C5
   |1C7
   |1D6
   |1D8
   |1E3
   |1E7
   |1E9
   |1F8
   |1G3
   |1G5
   |1G7
   |1G9
   |1H4
   |1H6
   |1H8
   |1H10
   |1J2
   |1J5
   |1J7
   |1J9
F7   | 41   VPP   F7
B5   | 42   ATEST0   B5
Y19   | 43   ATEST1   Y19
Y13   | 44   CSI0_ATB_0_H   Y13
Y14   | 45   CSI0_ATB_1_H   Y14
AE12   | 46   CSI0_RXCLKN   AE12
AE11   | 47   CSI0_RXCLKP   AE11
AB11   | 48   CSI0_RXN0   AB11
AC10   | 49   CSI0_RXN1   AC10
AA10   | 50   CSI0_RXN2   AA10
AD9   | 51   CSI0_RXN3   AD9
AB10   | 52   CSI0_RXP0   AB10
AC9   | 53   CSI0_RXP1   AC9
AA9   | 54   CSI0_RXP2   AA9
AD8   | 55   CSI0_RXP3   AD8
AA15   | 56   CSI0_RXRCALIB   AA15
K5   | 57   DDR0_A0   K5
L2   | 58   DDR0_A1   L2
L3   | 59   DDR0_A2   L3
M2   | 60   DDR0_A3   M2
N2   | 61   DDR0_A4   N2
K2   | 62   DDR0_A5   K2
N3   | 63   DDR0_A6   N3
L1   | 64   DDR0_A7   L1
M1   | 65   DDR0_A8   M1
T2   | 66   DDR0_A9   T2
R2   | 67   DDR0_A10   R2
N5   | 68   DDR0_A11   N5
P3   | 69   DDR0_A12   P3
P2   | 70   DDR0_A13   P2
T6   | 71   DDR0_ACT_N   T6
K3   | 72   DDR0_ALERT_N   K3
H5   | 73   DDR0_ATB0   H5
K6   | 74   DDR0_ATB1   K6
N6   | 75   DDR0_BA0   N6
K4   | 76   DDR0_BA1   K4
Y6   | 77   DDR0_BG0   Y6
U6   | 78   DDR0_BG1   U6
Y5   | 79   DDR0_CAL0   Y5
T5   | 80   DDR0_CAS_N   T5
R1   | 81   DDR0_CK0   R1
P1   | 82   DDR0_CK0_N   P1
N4   | 83   DDR0_CKE0   N4
P5   | 84   DDR0_CKE1   P5
L6   | 85   DDR0_CS0_N   L6
T3   | 86   DDR0_CS1_N   T3
C3   | 87   DDR0_DM0   C3
H3   | 88   DDR0_DM1   H3
V4   | 89   DDR0_DM2   V4
AD1   | 90   DDR0_DM3   AD1
B2   | 91   DDR0_DQ0   B2
A3   | 92   DDR0_DQ1   A3
A4   | 93   DDR0_DQ2   A4
A5   | 94   DDR0_DQ3   A5
A2   | 95   DDR0_DQ4   A2
B4   | 96   DDR0_DQ5   B4
D2   | 97   DDR0_DQ6   D2
C4   | 98   DDR0_DQ7   C4
E2   | 99   DDR0_DQ8   E2
F1   | 100   DDR0_DQ9   F1
G5   | 101   DDR0_DQ10   G5
F2   | 102   DDR0_DQ11   F2
G3   | 103   DDR0_DQ12   G3
H4   | 104   DDR0_DQ13   H4
J2   | 105   DDR0_DQ14   J2
G2   | 106   DDR0_DQ15   G2
U2   | 107   DDR0_DQ16   U2
U3   | 108   DDR0_DQ17   U3
U5   | 109   DDR0_DQ18   U5
V5   | 110   DDR0_DQ19   V5
V2   | 111   DDR0_DQ20   V2
Y2   | 112   DDR0_DQ21   Y2
Y3   | 113   DDR0_DQ22   Y3
AA4   | 114   DDR0_DQ23   AA4
AC2   | 115   DDR0_DQ24   AC2
AA2   | 116   DDR0_DQ25   AA2
AC4   | 117   DDR0_DQ26   AC4
AD2   | 118   DDR0_DQ27   AD2
AD3   | 119   DDR0_DQ28   AD3
AC3   | 120   DDR0_DQ29   AC3
AE4   | 121   DDR0_DQ30   AE4
AE3   | 122   DDR0_DQ31   AE3
D1   | 123   DDR0_DQS0   D1
C1   | 124   DDR0_DQS0_N   C1
J1   | 125   DDR0_DQS1   J1
H1   | 126   DDR0_DQS1_N   H1
W1   | 127   DDR0_DQS2   W1
V1   | 128   DDR0_DQS2_N   V1
AA1   | 129   DDR0_DQS3   AA1
AB1   | 130   DDR0_DQS3_N   AB1
L5   | 131   DDR0_ODT0   L5
V6   | 132   DDR0_ODT1   V6
T1   | 133   DDR0_PAR   T1
P6   | 134   DDR0_RAS_N   P6
AA5   | 135   DDR0_RESET0_N   AA5
T4   | 136   DDR0_WE_N   T4
AA17   | 137   DSI0_ATB_0_H   AA17
Y17   | 138   DSI0_ATB_1_H   Y17
AA12   | 139   DSI0_TXCLKN   AA12
AA13   | 140   DSI0_TXCLKP   AA13
AD11   | 141   DSI0_TXN0   AD11
AB13   | 142   DSI0_TXN1   AB13
AC12   | 143   DSI0_TXN2   AC12
AE14   | 144   DSI0_TXN3   AE14
AD12   | 145   DSI0_TXP0   AD12
AB14   | 146   DSI0_TXP1   AB14
AC13   | 147   DSI0_TXP2   AC13
AE15   | 148   DSI0_TXP3   AE15
Y16   | 149   DSI0_TXRCALIB   Y16
B12   | 150   EMU0   B12
D13   | 151   EMU1   D13
C23   | 152   EXTINTN   C23
C25   | 153   EXT_REFCLK1   C25
U22   | 154   GPMC0_AD0   U22
U21   | 155   GPMC0_AD1   U21
U20   | 156   GPMC0_AD2   U20
V25   | 157   GPMC0_AD3   V25
T20   | 158   GPMC0_AD4   T20
T21   | 159   GPMC0_AD5   T21
V24   | 160   GPMC0_AD6   V24
W25   | 161   GPMC0_AD7   W25
AC25   | 162   GPMC0_AD8   AC25
AB25   | 163   GPMC0_AD9   AB25
AA25   | 164   GPMC0_AD10   AA25
W24   | 165   GPMC0_AD11   W24
Y24   | 166   GPMC0_AD12   Y24
AD25   | 167   GPMC0_AD13   AD25
AB24   | 168   GPMC0_AD14   AB24
AC24   | 169   GPMC0_AD15   AC24
R25   | 170   GPMC0_ADVN_ALE   R25
U24   | 171   GPMC0_BE0N_CLE   U24
T24   | 172   GPMC0_BE1N   T24
Y25   | 173   GPMC0_CLK   Y25
T23   | 174   GPMC0_CSN0   T23
U23   | 175   GPMC0_CSN1   U23
T22   | 176   GPMC0_CSN2   T22
U25   | 177   GPMC0_CSN3   U25
P25   | 178   GPMC0_DIR   P25
R24   | 179   GPMC0_OEN_REN   R24
AA24   | 180   GPMC0_WAIT0   AA24
AD24   | 181   GPMC0_WAIT1   AD24
T25   | 182   GPMC0_WEN   T25
P24   | 183   GPMC0_WPN   P24
B25   | 184   I2C0_SCL   B25
A24   | 185   I2C0_SDA   A24
C24   | 186   I2C1_SCL   C24
B24   | 187   I2C1_SDA   B24
C5   | 188   IFORCE   C5
F20   | 189   MCAN0_RX   F20
B23   | 190   MCAN0_TX   B23
G20   | 191   MCASP0_ACLKR   G20
F24   | 192   MCASP0_ACLKX   F24
G23   | 193   MCASP0_AFSR   G23
F25   | 194   MCASP0_AFSX   F25
F23   | 195   MCASP0_AXR0   F23
E24   | 196   MCASP0_AXR1   E24
E25   | 197   MCASP0_AXR2   E25
D25   | 198   MCASP0_AXR3   D25
G6   | 199   MCU_ERRORN   G6
E11   | 200   MCU_I2C0_SCL   E11
D11   | 201   MCU_I2C0_SDA   D11
D6   | 202   MCU_MCAN0_RX   D6
E8   | 203   MCU_MCAN0_TX   E8
E7   | 204   MCU_MCAN1_RX   E7
F8   | 205   MCU_MCAN1_TX   F8
A10   | 206   MCU_OSC0_XI   A10
A11   | 207   MCU_OSC0_XO   A11
H6   | 208   MCU_PORZ   H6
F14   | 209   MCU_RESETSTATZ   F14
F11   | 210   MCU_RESETZ   F11
C10   | 211   MCU_SPI0_CLK   C10
B10   | 212   MCU_SPI0_CS0   B10
E10   | 213   MCU_SPI0_CS1   E10
B11   | 214   MCU_SPI0_D0   B11
D10   | 215   MCU_SPI0_D1   D10
B8   | 216   MCU_UART0_CTSN   B8
B7   | 217   MCU_UART0_RTSN   B7
B6   | 218   MCU_UART0_RXD   B6
C8   | 219   MCU_UART0_TXD   C8
F17   | 220   MDIO0_MDC   F17
F16   | 221   MDIO0_MDIO   F16
AC5   | 222   MMC0_CALPAD   AC5
AA6   | 223   MMC0_CLK   AA6
AB8   | 224   MMC0_CMD   AB8
AC7   | 225   MMC0_DAT0   AC7
AB7   | 226   MMC0_DAT1   AB7
AD6   | 227   MMC0_DAT2   AD6
AE5   | 228   MMC0_DAT3   AE5
AE6   | 229   MMC0_DAT4   AE6
AC6   | 230   MMC0_DAT5   AC6
AA7   | 231   MMC0_DAT6   AA7
AB6   | 232   MMC0_DAT7   AB6
AD5   | 233   MMC0_DS   AD5
J24   | 234   MMC1_CLK   J24
H20   | 235   MMC1_CMD   H20
H21   | 236   MMC1_DAT0   H21
H23   | 237   MMC1_DAT1   H23
H22   | 238   MMC1_DAT2   H22
H25   | 239   MMC1_DAT3   H25
D23   | 240   MMC1_SDCD   D23
D24   | 241   MMC1_SDWP   D24
K21   | 242   MMC2_CLK   K21
K24   | 243   MMC2_CMD   K24
K23   | 244   MMC2_DAT0   K23
K22   | 245   MMC2_DAT1   K22
L20   | 246   MMC2_DAT2   L20
L21   | 247   MMC2_DAT3   L21
J25   | 248   MMC2_SDCD   J25
K25   | 249   MMC2_SDWP   K25
AE20   | 250   OLDI0_A0N   AE20
AD20   | 251   OLDI0_A0P   AD20
AC19   | 252   OLDI0_A1N   AC19
AD19   | 253   OLDI0_A1P   AD19
AA19   | 254   OLDI0_A2N   AA19
AB19   | 255   OLDI0_A2P   AB19
AD18   | 256   OLDI0_A3N   AD18
AE19   | 257   OLDI0_A3P   AE19
AD17   | 258   OLDI0_A4N   AD17
AD16   | 259   OLDI0_A4P   AD16
AB17   | 260   OLDI0_A5N   AB17
AC17   | 261   OLDI0_A5P   AC17
AC16   | 262   OLDI0_A6N   AC16
AC15   | 263   OLDI0_A6P   AC15
AB16   | 264   OLDI0_A7N   AB16
AA16   | 265   OLDI0_A7P   AA16
AE18   | 266   OLDI0_CLK0N   AE18
AE17   | 267   OLDI0_CLK0P   AE17
AD15   | 268   OLDI0_CLK1N   AD15
AD14   | 269   OLDI0_CLK1P   AD14
P23   | 270   OSPI0_CLK   P23
M25   | 271   OSPI0_CSN0   M25
L24   | 272   OSPI0_CSN1   L24
L22   | 273   OSPI0_CSN2   L22
L23   | 274   OSPI0_CSN3   L23
L25   | 275   OSPI0_D0   L25
N24   | 276   OSPI0_D1   N24
N25   | 277   OSPI0_D2   N25
M24   | 278   OSPI0_D3   M24
N21   | 279   OSPI0_D4   N21
N22   | 280   OSPI0_D5   N22
P21   | 281   OSPI0_D6   P21
N20   | 282   OSPI0_D7   N20
P22   | 283   OSPI0_DQS   P22
N23   | 284   OSPI0_LBCLKO   N23
B9   | 285   PMIC_LPM_EN0   B9
H24   | 286   PORZ_OUT   H24
G25   | 287   RESETSTATZ   G25
G24   | 288   RESET_REQZ   G24
B15   | 289   RGMII1_RD0   B15
B16   | 290   RGMII1_RD1   B16
A14   | 291   RGMII1_RD2   A14
B14   | 292   RGMII1_RD3   B14
A16   | 293   RGMII1_RXC   A16
A15   | 294   RGMII1_RX_CTL   A15
A18   | 295   RGMII1_TD0   A18
C17   | 296   RGMII1_TD1   C17
A17   | 297   RGMII1_TD2   A17
C16   | 298   RGMII1_TD3   C16
B17   | 299   RGMII1_TXC   B17
B18   | 300   RGMII1_TX_CTL   B18
E19   | 301   RGMII2_RD0   E19
E16   | 302   RGMII2_RD1   E16
E17   | 303   RGMII2_RD2   E17
C19   | 304   RGMII2_RD3   C19
D19   | 305   RGMII2_RXC   D19
F19   | 306   RGMII2_RX_CTL   F19
B19   | 307   RGMII2_TD0   B19
A21   | 308   RGMII2_TD1   A21
D17   | 309   RGMII2_TD2   D17
A19   | 310   RGMII2_TD3   A19
D16   | 311   RGMII2_TXC   D16
A20   | 312   RGMII2_TX_CTL   A20
B21   | 313   SPI0_CLK   B21
D20   | 314   SPI0_CS0   D20
E20   | 315   SPI0_CS1   E20
B20   | 316   SPI0_D0   B20
C21   | 317   SPI0_D1   C21
C13   | 318   TCK   C13
E13   | 319   TDI   E13
C14   | 320   TDO   C14
F10   | 321   TEMP_DIODE_P   F10
E14   | 322   TMS   E14
B13   | 323   TRSTN   B13
A23   | 324   UART0_CTSN   A23
C22   | 325   UART0_RTSN   C22
A22   | 326   UART0_RXD   A22
B22   | 327   UART0_TXD   B22
AE8   | 328   USB0_DM   AE8
AE7   | 329   USB0_DP   AE7
G22   | 330   USB0_DRVVBUS   G22
Y8   | 331   USB0_RCALIB   Y8
Y7   | 332   USB0_VBUS   Y7
AE10   | 333   USB1_DM   AE10
AE9   | 334   USB1_DP   AE9
G21   | 335   USB1_DRVVBUS   G21
1K4   | 336   USB1_RCALIB   1K4
Y10   | 337   USB1_VBUS   Y10
1A10   | 338   VMON_1P8_SOC   1A10
1A4   | 339   VMON_3P3_SOC   1A4
1A6   | 340   VMON_ER_VSYS   1A6
AE24   | 341   VOUT0_DATA0   AE24
W23   | 342   VOUT0_DATA1   W23
AA23   | 343   VOUT0_DATA2   AA23
Y23   | 344   VOUT0_DATA3   Y23
AB23   | 345   VOUT0_DATA4   AB23
AD23   | 346   VOUT0_DATA5   AD23
AC23   | 347   VOUT0_DATA6   AC23
AE23   | 348   VOUT0_DATA7   AE23
AE22   | 349   VOUT0_DATA8   AE22
AC22   | 350   VOUT0_DATA9   AC22
W22   | 351   VOUT0_DATA10   W22
AE21   | 352   VOUT0_DATA11   AE21
AD21   | 353   VOUT0_DATA12   AD21
AC21   | 354   VOUT0_DATA13   AC21
AA20   | 355   VOUT0_DATA14   AA20
Y20   | 356   VOUT0_DATA15   Y20
W21   | 357   VOUT0_DE   W21
AC20   | 358   VOUT0_HSYNC   AC20
Y21   | 359   VOUT0_PCLK   Y21
W20   | 360   VOUT0_VSYNC   W20
F6   | 361   VSENSE   F6
F13   | 362   WKUP_CLKOUT0   F13
A13   | 363   WKUP_I2C0_SCL   A13
C11   | 364   WKUP_I2C0_SDA   C11
A7   | 365   WKUP_LFOSC0_XI   A7
A8   | 366   WKUP_LFOSC0_XO   A8
C7   | 367   WKUP_UART0_CTSN   C7
C6   | 368   WKUP_UART0_RTSN   C6
D8   | 369   WKUP_UART0_RXD   D8
D7   | 370   WKUP_UART0_TXD   D7
[Model Data]
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[End Model Data]
[End Package Model]
| Models and submodels in the file (204): lvcmos1_nom_1p8_h (I/O), lvcmos0_nom_1p8_v (I/O), lvcmos1_nom_3p3_h (I/O), lvcmos0_nom_3p3_v (I/O), lvcmos1_slow_1p8_h (I/O), lvcmos0_slow_1p8_v (I/O), lvcmos1_slow_3p3_h (I/O), lvcmos0_slow_3p3_v (I/O), lvcmos1_fast_1p8_h (I/O), lvcmos0_fast_1p8_v (I/O), lvcmos1_fast_3p3_h (I/O), lvcmos0_fast_3p3_v (I/O), sdio1_r33_1p8_h (I/O), sdio0_r33_1p8_v (I/O), sdio1_r33_3p3_h (I/O), sdio0_r33_3p3_v (I/O), sdio1_r40_1p8_h (I/O), sdio0_r40_1p8_v (I/O), sdio1_r40_3p3_h (I/O), sdio0_r40_3p3_v (I/O), sdio1_r50_1p8_h (I/O), sdio0_r50_1p8_v (I/O), sdio1_r50_3p3_h (I/O), sdio0_r50_3p3_v (I/O), sdio1_r66_1p8_h (I/O), sdio0_r66_1p8_v (I/O), sdio1_r66_3p3_h (I/O), sdio0_r66_3p3_v (I/O), lpddr4_ocd_40p_40n_lt (I/O), lpddr4_ocd_48p_48n_lt (I/O), lpddr4_ocd_60p_60n_lt (I/O), lpddr4_ocd_60p_60n_120pd_lt (I/O), lpddr4_ocd_80p_80n_lt (I/O), lpddr4_ocd_40p_40n_p_lt (I/O), lpddr4_ocd_40p_40n_n_lt (I/O), lpddr4_ocd_48p_48n_p_lt (I/O), lpddr4_ocd_48p_48n_n_lt (I/O), lpddr4_ocd_60p_60n_p_lt (I/O), lpddr4_ocd_60p_60n_n_lt (I/O), lpddr4_ocd_60p_60n_120pd_p_lt (I/O), lpddr4_ocd_60p_60n_120pd_n_lt (I/O), lpddr4_ocd_80p_80n_p_lt (I/O), lpddr4_ocd_80p_80n_n_lt (I/O), lpddr4_odt_40_lt (Input), lpddr4_odt_48_lt (Input), lpddr4_odt_60_lt (Input), lpddr4_odt_80_lt (Input), lpddr4_odt_120_lt (Input), lpddr4_odt_240_lt (Input), lpddr4_odt_off_lt (Input), lpddr4_odt_40_diff_lt (Input), lpddr4_odt_48_diff_lt (Input), lpddr4_odt_60_diff_lt (Input), lpddr4_odt_80_diff_lt (Input), lpddr4_odt_120_diff_lt (Input), lpddr4_odt_240_diff_lt (Input), lpddr4_odt_off_diff_lt (Input), lpddr4_ocd_40p_40n_ht (I/O), lpddr4_ocd_48p_48n_ht (I/O), lpddr4_ocd_60p_60n_ht (I/O), lpddr4_ocd_60p_60n_120pd_ht (I/O), lpddr4_ocd_80p_80n_ht (I/O), lpddr4_ocd_40p_40n_p_ht (I/O), lpddr4_ocd_40p_40n_n_ht (I/O), lpddr4_ocd_48p_48n_p_ht (I/O), lpddr4_ocd_48p_48n_n_ht (I/O), lpddr4_ocd_60p_60n_p_ht (I/O), lpddr4_ocd_60p_60n_n_ht (I/O), lpddr4_ocd_60p_60n_120pd_p_ht (I/O), lpddr4_ocd_60p_60n_120pd_n_ht (I/O), lpddr4_ocd_80p_80n_p_ht (I/O), lpddr4_ocd_80p_80n_n_ht (I/O), lpddr4_odt_40_ht (Input), lpddr4_odt_48_ht (Input), lpddr4_odt_60_ht (Input), lpddr4_odt_80_ht (Input), lpddr4_odt_120_ht (Input), lpddr4_odt_240_ht (Input), lpddr4_odt_off_ht (Input), lpddr4_odt_40_diff_ht (Input)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
